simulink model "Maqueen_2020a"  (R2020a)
settings: Solver=VariableStepAuto  StartTime=0.0  StopTime=2  RelTol=1e-3
model workspace: external: MAT-File (data not in the file)
undefined symbols (not defined in the file or in its folder): deg, kg, m, mm, N, rad, s, smiData, X, Y, Z
libraries: sm_lib x459, fl_lib x12, nesl_utility x10
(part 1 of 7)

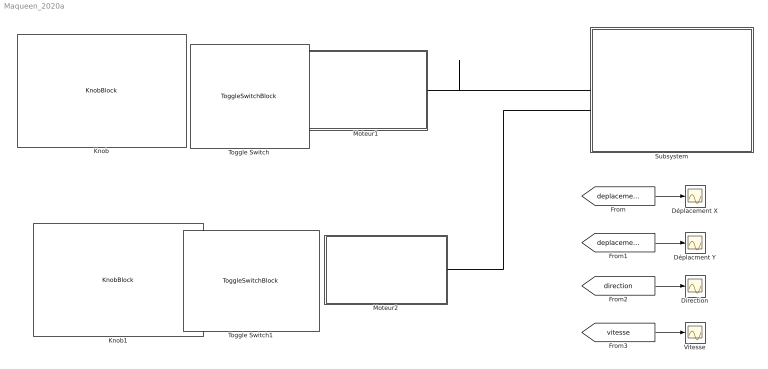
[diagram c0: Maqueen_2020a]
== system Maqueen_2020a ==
  Direction : Scope
  Déplacement X : Scope
  Déplacment Y : Scope
  Knob : KnobBlock  ScaleMax=255
  Knob1 : KnobBlock  ScaleMax=255
  Moteur1 : Subsystem
  Moteur2 : Subsystem
  Subsystem : Subsystem
  Toggle Switch : ToggleSwitchBlock
  Toggle Switch1 : ToggleSwitchBlock
  Vitesse : Scope
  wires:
  [deplacementX] -> Déplacement X/1
  [vitesse] -> Vitesse/1
  [direction] -> Direction/1
  [deplacementY] -> Déplacment Y/1
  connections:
  Moteur2/RConn1 -- Subsystem/LConn2
  Moteur1/RConn1 -- Subsystem/LConn1

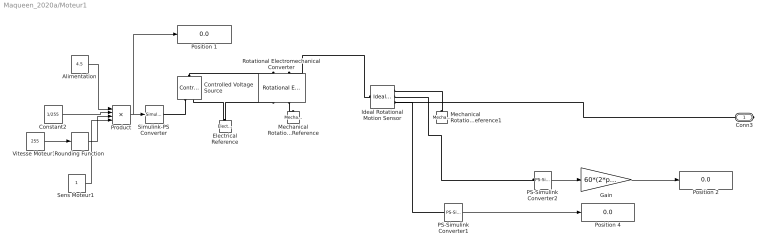
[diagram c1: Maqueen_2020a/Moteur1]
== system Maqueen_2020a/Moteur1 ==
  Alimentation : Constant  Value=4.5
  Constant2 : Constant  Value=1/255
  Controlled Voltage Source : fl_lib/Electrical/Electrical Sources/Controlled Voltage Source
  Electrical Reference : fl_lib/Electrical/Electrical Elements/Electrical Reference
  Gain : Gain  Gain=60*(2*pi)
  Ideal Rotational Motion Sensor : fl_lib/Mechanical/Mechanical Sensors/Ideal Rotational Motion Sensor  wrap_angle=simscape.enum.onoff.off  offset=0 rad
  Mechanical Rotational Reference : fl_lib/Mechanical/Rotational Elements/Mechanical Rotational Reference
  Mechanical Rotational Reference1 : fl_lib/Mechanical/Rotational Elements/Mechanical Rotational Reference
  PS-Simulink Converter1 : nesl_utility/PS-Simulink Converter  PhysicalDomain=network_engine_domain  SubClassName=ps_output  LeftPortType=input  RightPortType=output  PseudoPeriodic=off  Frequencies=[]  Unit=1  AffineConversion=off
  PS-Simulink Converter2 : nesl_utility/PS-Simulink Converter  PhysicalDomain=network_engine_domain  SubClassName=ps_output  LeftPortType=input  RightPortType=output  PseudoPeriodic=off  Frequencies=[]  Unit=1  AffineConversion=off
  Position 1 : Display
  Position 2 : Display
  Position 4 : Display
  Product : Product  Inputs=4
  Rotational Electromechanical Converter : fl_lib/Electrical/Electrical Elements/Rotational Electromechanical Converter  K=4.5/85.5 V/rpm  i_specify=off  i_priority=None  i=0 A  i_nominal_specify=off  i_nominal_unit=A  i_nominal_value=1  v_specify=off  v_priority=None  v=0 V  v_nominal_specify=off  v_nominal_unit=V  v_nominal_value=1  t_specify=off  t_priority=None  t=0 N*m  t_nominal_specify=off  t_nominal_unit=N*m  t_nominal_value=1  w_specify=off  w_priority=None  w=0 rad/s  w_nominal_specify=off  w_nominal_unit=rad/s  w_nominal_value=1
  Rounding Function : Rounding
  "Sens Moteur1 " : Constant
  Simulink-PS Converter : nesl_utility/Simulink-PS Converter  PhysicalDomain=network_engine_domain  SubClassName=ps_input  LeftPortType=input  RightPortType=output  PseudoPeriodic=off  Frequencies=[]  NoiseDistribution=none  NoiseParameters=[]  Unit=1  AffineConversion=off  FilteringAndDerivatives=provide  SimscapeFilterOrder=1  InputFilterTimeConstant=0.001  UdotUserProvided=0
  "Vitesse Moteur1 " : Constant  Value=255
  Conn3 : PMIOPort  Side=Right
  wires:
  "Sens Moteur1 "/1 -> Product/4
  Product/1 -> Position 1/1, Simulink-PS Converter/1
  "Vitesse Moteur1 "/1 -> Rounding Function/1
  Alimentation/1 -> Product/1
  Constant2/1 -> Product/2
  Rounding Function/1 -> Product/3
  PS-Simulink Converter2/1 -> Gain/1
  Gain/1 -> Position 2/1
  PS-Simulink Converter1/1 -> Position 4/1
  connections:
  Electrical Reference/LConn1 -- Rotational Electromechanical Converter/RConn1 -- Controlled Voltage Source/RConn2
  Rotational Electromechanical Converter/RConn2 -- Mechanical Rotational Reference/LConn1
  Ideal Rotational Motion Sensor/LConn1 -- Rotational Electromechanical Converter/LConn2
  Mechanical Rotational Reference1/LConn1 -- Ideal Rotational Motion Sensor/RConn1
  Controlled Voltage Source/RConn1 -- Simulink-PS Converter/RConn1
  Ideal Rotational Motion Sensor/RConn3 -- Conn3/RConn1 -- PS-Simulink Converter1/LConn1
  Controlled Voltage Source/LConn1 -- Rotational Electromechanical Converter/LConn1
  PS-Simulink Converter2/LConn1 -- Ideal Rotational Motion Sensor/RConn2

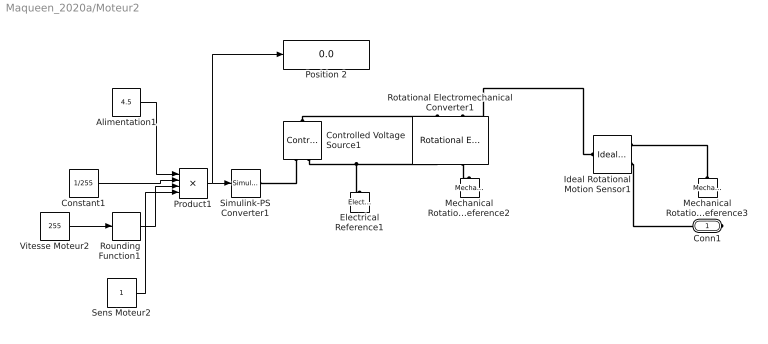
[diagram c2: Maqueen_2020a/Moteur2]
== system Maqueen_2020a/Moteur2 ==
  Alimentation1 : Constant  Value=4.5
  Constant1 : Constant  Value=1/255
  Controlled Voltage Source1 : fl_lib/Electrical/Electrical Sources/Controlled Voltage Source
  Electrical Reference1 : fl_lib/Electrical/Electrical Elements/Electrical Reference
  Ideal Rotational Motion Sensor1 : fl_lib/Mechanical/Mechanical Sensors/Ideal Rotational Motion Sensor  wrap_angle=simscape.enum.onoff.off  offset=0 rad
  Mechanical Rotational Reference2 : fl_lib/Mechanical/Rotational Elements/Mechanical Rotational Reference
  Mechanical Rotational Reference3 : fl_lib/Mechanical/Rotational Elements/Mechanical Rotational Reference
  Position 2 : Display
  Product1 : Product  Inputs=4
  Rotational Electromechanical Converter1 : fl_lib/Electrical/Electrical Elements/Rotational Electromechanical Converter  K=4.5/85.5 V/rpm  i_specify=off  i_priority=None  i=0 A  i_nominal_specify=off  i_nominal_unit=A  i_nominal_value=1  v_specify=off  v_priority=None  v=0 V  v_nominal_specify=off  v_nominal_unit=V  v_nominal_value=1  t_specify=off  t_priority=None  t=0 N*m  t_nominal_specify=off  t_nominal_unit=N*m  t_nominal_value=1  w_specify=off  w_priority=None  w=0 rad/s  w_nominal_specify=off  w_nominal_unit=rad/s  w_nominal_value=1
  Rounding Function1 : Rounding
  Sens Moteur2 : Constant
  Simulink-PS Converter1 : nesl_utility/Simulink-PS Converter  PhysicalDomain=network_engine_domain  SubClassName=ps_input  LeftPortType=input  RightPortType=output  PseudoPeriodic=off  Frequencies=[]  NoiseDistribution=none  NoiseParameters=[]  Unit=1  AffineConversion=off  FilteringAndDerivatives=provide  SimscapeFilterOrder=1  InputFilterTimeConstant=0.001  UdotUserProvided=0
  Vitesse Moteur2 : Constant  Value=255
  Conn1 : PMIOPort  Side=Right
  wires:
  Vitesse Moteur2/1 -> Rounding Function1/1
  Alimentation1/1 -> Product1/1
  Sens Moteur2/1 -> Product1/4
  Product1/1 -> Position 2/1, Simulink-PS Converter1/1
  Rounding Function1/1 -> Product1/3
  Constant1/1 -> Product1/2
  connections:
  Ideal Rotational Motion Sensor1/RConn3 -- Conn1/RConn1
  Controlled Voltage Source1/RConn1 -- Simulink-PS Converter1/RConn1
  Rotational Electromechanical Converter1/RConn2 -- Mechanical Rotational Reference2/LConn1
  Controlled Voltage Source1/RConn2 -- Rotational Electromechanical Converter1/RConn1 -- Electrical Reference1/LConn1
  Ideal Rotational Motion Sensor1/LConn1 -- Rotational Electromechanical Converter1/LConn2
  Mechanical Rotational Reference3/LConn1 -- Ideal Rotational Motion Sensor1/RConn1
  Controlled Voltage Source1/LConn1 -- Rotational Electromechanical Converter1/LConn1

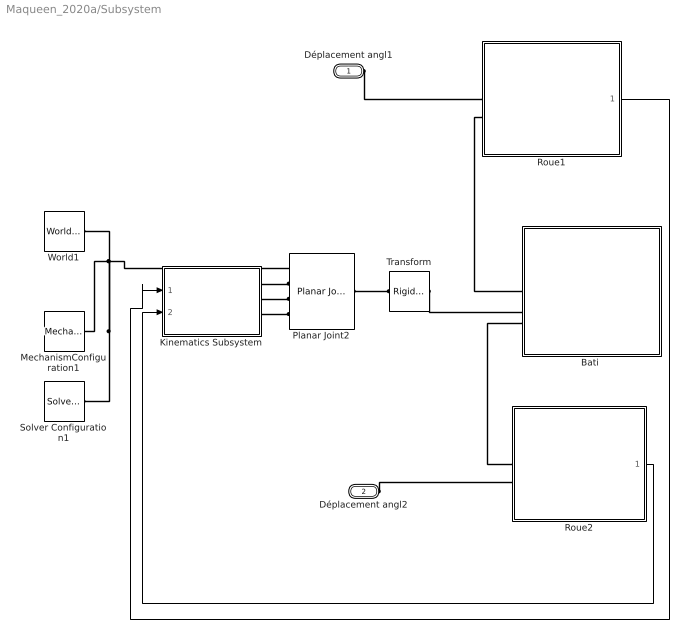
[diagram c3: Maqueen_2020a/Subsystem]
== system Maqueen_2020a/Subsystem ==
  "Bati " : Subsystem
  Kinematics Subsystem : Subsystem
  MechanismConfiguration1 : sm_lib/Utilities/Mechanism Configuration  UniformGravity=Constant  GravityVector=[0 0 -9.80665]  GravityUnits=m/s^2  LinearizationDelta=0.001
  Planar Joint2 : sm_lib/Joints/Planar Joint  JointMode=Normal  SenseConstraintForce=off  SenseConstraintForceX=off  SenseConstraintForceY=off  SenseConstraintForceZ=off  SenseConstraintTorque=off  SenseConstraintTorqueX=off  SenseConstraintTorqueY=off  SenseConstraintTorqueZ=off  SenseTotalForce=off  SenseTotalForceX=off  SenseTotalForceY=off  SenseTotalForceZ=off  SenseTotalTorque=off  SenseTotalTorqueX=off  SenseTotalTorqueY=off  SenseTotalTorqueZ=off  CompositeWrenchDir=FollowerOnBase  CompositeWrenchFrame=BaseFrame  PxEquilibriumPosition=0  PxEquilibriumPositionUnits=m  PxSpringStiffness=0  PxSpringStiffnessUnits=N/m  PxDampingCoefficient=0  PxDampingCoefficientUnits=N/(m/s)  PxTorqueActuationMode=ComputedTorque  PxMotionActuationMode=InputMotion  PxSensePosition=off  PxSenseVelocity=off  PxSenseAcceleration=off  PxSenseTorqueForce=off  PxSenseLowerLimitTorqueForce=off  PxSenseUpperLimitTorqueForce=off  PxLowerLimitSpecify=off  PxLowerLimitBound=-1  PxLowerLimitBoundUnits=m  PxLowerLimitStiffness=1e6  PxLowerLimitStiffnessUnits=N/m  PxLowerLimitDamping=1e3  PxLowerLimitDampingUnits=N/(m/s)  PxLowerLimitTransitionRegionWidth=1e-4  PxLowerLimitTransitionRegionWidthUnits=m  PxUpperLimitSpecify=off  PxUpperLimitBound=1  PxUpperLimitBoundUnits=m  PxUpperLimitStiffness=1e6  PxUpperLimitStiffnessUnits=N/m  PxUpperLimitDamping=1e3  PxUpperLimitDampingUnits=N/(m/s)  PxUpperLimitTransitionRegionWidth=1e-4  PxUpperLimitTransitionRegionWidthUnits=m  PxPositionTargetSpecify=off  PxPositionTargetPriority=High  PxPositionTargetValue=0  PxPositionTargetValueUnits=m  PxVelocityTargetSpecify=off  PxVelocityTargetPriority=High  PxVelocityTargetValue=0  PxVelocityTargetValueUnits=m/s  PyEquilibriumPosition=0  PyEquilibriumPositionUnits=m  PySpringStiffness=0  PySpringStiffnessUnits=N/m  PyDampingCoefficient=0  PyDampingCoefficientUnits=N/(m/s)  PyTorqueActuationMode=ComputedTorque  PyMotionActuationMode=InputMotion  PySensePosition=off  PySenseVelocity=off  PySenseAcceleration=off  PySenseTorqueForce=off  PySenseLowerLimitTorqueForce=off  PySenseUpperLimitTorqueForce=off  PyLowerLimitSpecify=off  PyLowerLimitBound=-1  PyLowerLimitBoundUnits=m  PyLowerLimitStiffness=1e6  PyLowerLimitStiffnessUnits=N/m  PyLowerLimitDamping=1e3  PyLowerLimitDampingUnits=N/(m/s)  PyLowerLimitTransitionRegionWidth=1e-4  PyLowerLimitTransitionRegionWidthUnits=m  PyUpperLimitSpecify=off  PyUpperLimitBound=1  PyUpperLimitBoundUnits=m  PyUpperLimitStiffness=1e6  PyUpperLimitStiffnessUnits=N/m  PyUpperLimitDamping=1e3  PyUpperLimitDampingUnits=N/(m/s)  PyUpperLimitTransitionRegionWidth=1e-4  PyUpperLimitTransitionRegionWidthUnits=m  PyPositionTargetSpecify=off  PyPositionTargetPriority=High  PyPositionTargetValue=0  PyPositionTargetValueUnits=m  PyVelocityTargetSpecify=off  PyVelocityTargetPriority=High  PyVelocityTargetValue=0  PyVelocityTargetValueUnits=m/s  RzEquilibriumPosition=0  RzEquilibriumPositionUnits=deg  RzSpringStiffness=0  RzSpringStiffnessUnits=N*m/deg  RzDampingCoefficient=0  RzDampingCoefficientUnits=N*m/(deg/s)  RzTorqueActuationMode=ComputedTorque  RzMotionActuationMode=InputMotion  RzSensePosition=off  RzSenseVelocity=off  RzSenseAcceleration=off  RzSenseTorqueForce=off  RzSenseLowerLimitTorqueForce=off  RzSenseUpperLimitTorqueForce=off  RzLowerLimitSpecify=off  RzLowerLimitBound=-90  RzLowerLimitBoundUnits=deg  RzLowerLimitStiffness=1e4  RzLowerLimitStiffnessUnits=N*m/deg  RzLowerLimitDamping=10  RzLowerLimitDampingUnits=N*m/(deg/s)  RzLowerLimitTransitionRegionWidth=0.1  RzLowerLimitTransitionRegionWidthUnits=deg  RzUpperLimitSpecify=off  RzUpperLimitBound=90  RzUpperLimitBoundUnits=deg  RzUpperLimitStiffness=1e4  RzUpperLimitStiffnessUnits=N*m/deg  RzUpperLimitDamping=10  RzUpperLimitDampingUnits=N*m/(deg/s)  RzUpperLimitTransitionRegionWidth=0.1  RzUpperLimitTransitionRegionWidthUnits=deg  RzPositionTargetSpecify=off  RzPositionTargetPriority=High  RzPositionTargetValue=0  RzPositionTargetValueUnits=deg  RzVelocityTargetSpecify=off  RzVelocityTargetPriority=High  RzVelocityTargetValue=0  RzVelocityTargetValueUnits=deg/s
  Roue1 : Subsystem
  Roue2 : Subsystem
  Solver Configuration1 : nesl_utility/Solver Configuration  PhysicalDomain=network_engine_domain  SubClassName=solver  LeftPortType=input  RightPortType=generic  Tones=[]  Harmonics=[]  SimulateNoise=off  Profile=off  UseLocalSampling=off  EnableSwitchedLinearOptims=on  FrequencyDomain=off  UseCCode=off  RelTol=0.001  AbsTol=1e-06  MinStep=1e-09  ToWorkspace=off  RevertToSquareIcSolve=off  NumHomotopyIterations=100  PhasorMode=off  PhasorModeNumHarmonics=1  DoDC=off  ResidualTolerance=1e-09  UseLocalSolver=off  LocalSolverChoice=NE_BACKWARD_EULER_ADVANCER  LocalSolverSampleTime=0.001  DoFixedCost=off  MaxNonlinIter=3  MaxModeIter=2  LinearAlgebra=Sparse  EquationFormulation=NE_TIME_EF  DelaysMemoryBudget=1024  AutomaticFiltering=on  FilteringTimeConstant=0.001  PartitionStorageMethod=AS_NEEDED  PartitionMemoryBudget=1024  PartitionMethod=FAST
  Transform : sm_lib/Frames and Transforms/Rigid Transform  TranslationMethod=Cartesian  TranslationStandardOffset=0  TranslationLengthUnit=mm  TranslationStandardAxis=+Z  TranslationCartesianOffset=smiData.RigidTransform(161).translation  TranslationROffset=0  TranslationROffsetUnits=m  TranslationZOffset=0  TranslationZOffsetUnits=m  TranslationThetaOffset=0  TranslationThetaOffsetUnits=deg  RotationMethod=ArbitraryAxis  RotationAngleUnits=rad  RotationStandardAxis=+Z  RotationAngle=smiData.RigidTransform(161).angle  RotationArbitraryAxis=smiData.RigidTransform(161).axis  FollAlignAxisA=+X  BaseAlignAxisA=+Y  FollAlignAxisB=+Y  BaseAlignAxisB=+Z  RotationSequenceAxes=FollowerAxes  RotationSequence=XYX  RotationSequenceAngles=[0 0 0]  RotationSequenceAnglesUnits=deg  RotationMatrix=[1 0 0; 0 1 0; 0 0 1]
  World1 : sm_lib/Frames and Transforms/World Frame
  Déplacement angl1 : PMIOPort  Side=Left
  Déplacement angl2 : PMIOPort  Port=2  Side=Left
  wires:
  Roue2/1(Out1) -> Kinematics Subsystem/2(w_r)
  Roue1/1(Out1) -> Kinematics Subsystem/1(w_l)
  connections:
  MechanismConfiguration1/RConn1 -- Solver Configuration1/RConn1 -- Planar Joint2/LConn1 -- World1/RConn1
  "Bati "/LConn1 -- Roue1/LConn2
  Transform/RConn1 -- "Bati "/LConn2
  "Bati "/LConn3 -- Roue2/LConn1
  Planar Joint2/RConn1 -- Transform/LConn1
  Kinematics Subsystem/RConn1 -- Planar Joint2/LConn2
  Kinematics Subsystem/RConn2 -- Planar Joint2/LConn3
  Kinematics Subsystem/RConn3 -- Planar Joint2/LConn4
  Déplacement angl2/RConn1 -- Roue2/LConn2
  Déplacement angl1/RConn1 -- Roue1/LConn1

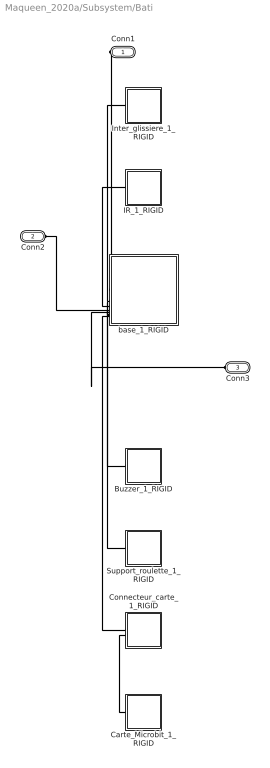
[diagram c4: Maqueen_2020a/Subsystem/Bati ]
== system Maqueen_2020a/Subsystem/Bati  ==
  Buzzer_1_RIGID : Subsystem
  Carte_Microbit_1_RIGID : Subsystem
  Connecteur_carte_1_RIGID : Subsystem
  IR_1_RIGID : Subsystem
  Inter_glissiere_1_RIGID : Subsystem
  Support_roulette_1_RIGID : Subsystem
  base_1_RIGID : Subsystem
  Conn1 : PMIOPort  Side=Left
  Conn2 : PMIOPort  Port=2  Side=Left
  Conn3 : PMIOPort  Port=3  Side=Left
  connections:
  base_1_RIGID/LConn1 -- Conn1/RConn1
  Support_roulette_1_RIGID/LConn1 -- base_1_RIGID/LConn7
  Connecteur_carte_1_RIGID/LConn1 -- base_1_RIGID/LConn8
  IR_1_RIGID/LConn1 -- base_1_RIGID/LConn3
  Carte_Microbit_1_RIGID/LConn1 -- Connecteur_carte_1_RIGID/LConn2
  Conn2/RConn1 -- base_1_RIGID/LConn4
  Inter_glissiere_1_RIGID/LConn1 -- base_1_RIGID/LConn2
  Buzzer_1_RIGID/LConn1 -- base_1_RIGID/LConn6
  base_1_RIGID/LConn5 -- Conn3/RConn1

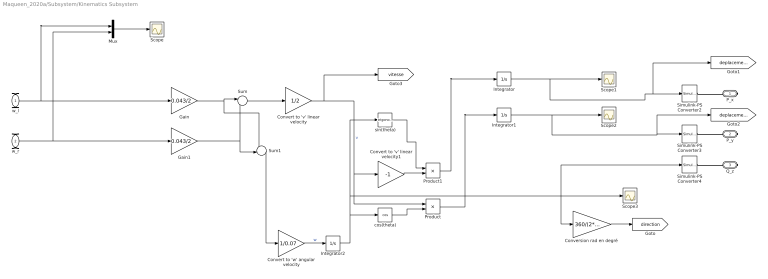
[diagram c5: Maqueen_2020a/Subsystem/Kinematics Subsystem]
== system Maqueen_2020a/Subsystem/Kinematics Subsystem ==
  w_l : Inport
  w_r : Inport  Port=2
  "Conversion rad en degré " : Gain  Gain=360/(2*pi)
  Convert to 'v' linear velocity : Gain  Gain=1/2
  Convert to 'v' linear velocity1 : Gain  Gain=-1
  Convert to 'w' angular velocity : Gain  Gain=1/0.07
  Gain : Gain  Gain=0.043/2
  Gain1 : Gain  Gain=0.043/2
  Integrator : Integrator
  Integrator1 : Integrator
  Integrator2 : Integrator
  Mux : Mux  Inputs=2
  Product : Product
  Product1 : Product
  Scope{,1..3} (4 alike) : Scope
  Simulink-PS Converter2 : nesl_utility/Simulink-PS Converter  PhysicalDomain=network_engine_domain  SubClassName=ps_input  LeftPortType=input  RightPortType=output  PseudoPeriodic=off  Frequencies=[]  NoiseDistribution=none  NoiseParameters=[]  Unit=1  AffineConversion=off  FilteringAndDerivatives=filter  SimscapeFilterOrder=2  InputFilterTimeConstant=0.01  UdotUserProvided=1
  Simulink-PS Converter3 : nesl_utility/Simulink-PS Converter  PhysicalDomain=network_engine_domain  SubClassName=ps_input  LeftPortType=input  RightPortType=output  PseudoPeriodic=off  Frequencies=[]  NoiseDistribution=none  NoiseParameters=[]  Unit=1  AffineConversion=off  FilteringAndDerivatives=filter  SimscapeFilterOrder=2  InputFilterTimeConstant=0.01  UdotUserProvided=1
  Simulink-PS Converter4 : nesl_utility/Simulink-PS Converter  PhysicalDomain=network_engine_domain  SubClassName=ps_input  LeftPortType=input  RightPortType=output  PseudoPeriodic=off  Frequencies=[]  NoiseDistribution=none  NoiseParameters=[]  Unit=1  AffineConversion=off  FilteringAndDerivatives=filter  SimscapeFilterOrder=2  InputFilterTimeConstant=0.01  UdotUserProvided=1
  Sum : Sum  Inputs=|++
  Sum1 : Sum  Inputs=-+|
  cos(theta) : Trigonometry  Operator=cos
  sin(theta) : Trigonometry
  P_x : PMIOPort  Side=Right
  P_y : PMIOPort  Port=2  Side=Right
  Q_z : PMIOPort  Port=3  Side=Right
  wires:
  Convert to 'v' linear velocity1/1 -> Product1/2
  Mux/1 -> Scope/1
  Product/1 -> Integrator1/1
  Product1/1 -> Integrator/1
  w_r/1 -> Gain1/1, Mux/2
  w_l/1 -> Gain/1, Mux/1
  Convert to 'v' linear velocity/1 -> [vitesse], Product/1, Convert to 'v' linear velocity1/1  "v"
  Sum1/1 -> Convert to 'w' angular velocity/1
  cos(theta)/1 -> Product/2
  sin(theta)/1 -> Product1/1
  Integrator2/1 -> cos(theta)/1, sin(theta)/1, Scope3/1, "Conversion rad en degré "/1, Simulink-PS Converter4/1
  Convert to 'w' angular velocity/1 -> Integrator2/1  "w"
  Integrator1/1 -> Scope2/1, [deplacementY], Simulink-PS Converter3/1
  Sum/1 -> Convert to 'v' linear velocity/1
  Gain/1 -> Sum/1, Sum1/1
  Gain1/1 -> Sum1/2, Sum/2
  "Conversion rad en degré "/1 -> [direction]
  Integrator/1 -> Scope1/1, [deplacementX], Simulink-PS Converter2/1
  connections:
  Simulink-PS Converter3/RConn1 -- P_y/RConn1
  Simulink-PS Converter2/RConn1 -- P_x/RConn1
  Simulink-PS Converter4/RConn1 -- Q_z/RConn1

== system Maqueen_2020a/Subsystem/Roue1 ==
  PS-Simulink Converter3 : nesl_utility/PS-Simulink Converter  PhysicalDomain=network_engine_domain  SubClassName=ps_output  LeftPortType=input  RightPortType=output  PseudoPeriodic=off  Frequencies=[]  Unit=1  AffineConversion=off
  Revolute : sm_lib/Joints/Revolute Joint  JointMode=Normal  SenseConstraintForce=off  SenseConstraintForceX=off  SenseConstraintForceY=off  SenseConstraintForceZ=off  SenseConstraintTorque=off  SenseConstraintTorqueX=off  SenseConstraintTorqueY=off  SenseConstraintTorqueZ=off  SenseTotalForce=off  SenseTotalForceX=off  SenseTotalForceY=off  SenseTotalForceZ=off  SenseTotalTorque=off  SenseTotalTorqueX=off  SenseTotalTorqueY=off  SenseTotalTorqueZ=off  CompositeWrenchDir=FollowerOnBase  CompositeWrenchFrame=BaseFrame  EquilibriumPosition=0  EquilibriumPositionUnits=rad  SpringStiffness=0  SpringStiffnessUnits=N*m/rad  DampingCoefficient=0  DampingCoefficientUnits=N*m/(rad/s)  TorqueActuationMode=ComputedTorque  MotionActuationMode=InputMotion  SensePosition=off  SenseVelocity=on  SenseAcceleration=off  SenseTorqueForce=off  SenseLowerLimitTorqueForce=off  SenseUpperLimitTorqueForce=off  LowerLimitSpecify=off  LowerLimitBound=-90  LowerLimitBoundUnits=deg  LowerLimitStiffness=1e4  LowerLimitStiffnessUnits=N*m/deg  LowerLimitDamping=10  LowerLimitDampingUnits=N*m/(deg/s)  LowerLimitTransitionRegionWidth=0.1  LowerLimitTransitionRegionWidthUnits=deg  UpperLimitSpecify=off  UpperLimitBound=90  UpperLimitBoundUnits=deg  UpperLimitStiffness=1e4  UpperLimitStiffnessUnits=N*m/deg  UpperLimitDamping=10  UpperLimitDampingUnits=N*m/(deg/s)  UpperLimitTransitionRegionWidth=0.1  UpperLimitTransitionRegionWidthUnits=deg  PositionTargetSpecify=on  PositionTargetPriority=Low  PositionTargetValue=smiData.RevoluteJoint(1).Rz.Pos  PositionTargetValueUnits=deg  VelocityTargetSpecify=off  VelocityTargetPriority=High  VelocityTargetValue=0  VelocityTargetValueUnits=deg/s
  Roue_2_RIGID : Subsystem
  bloc_moteur_1_RIGID : Subsystem
  Conn1 : PMIOPort  Side=Left
  Conn2 : PMIOPort  Port=2  Side=Left
  Out1 : Outport  VectorParamsAs1DForOutWhenUnconnected=off
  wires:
  PS-Simulink Converter3/1 -> Out1/1
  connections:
  Revolute/LConn2 -- Conn1/RConn1
  Revolute/LConn1 -- Roue_2_RIGID/RConn1
  Revolute/RConn1 -- bloc_moteur_1_RIGID/LConn1
  Conn2/RConn1 -- bloc_moteur_1_RIGID/LConn2
  Revolute/RConn2 -- PS-Simulink Converter3/LConn1

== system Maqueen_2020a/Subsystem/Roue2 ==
  PS-Simulink Converter1 : nesl_utility/PS-Simulink Converter  PhysicalDomain=network_engine_domain  SubClassName=ps_output  LeftPortType=input  RightPortType=output  PseudoPeriodic=off  Frequencies=[]  Unit=1  AffineConversion=off
  Revolute1 : sm_lib/Joints/Revolute Joint  JointMode=Normal  SenseConstraintForce=off  SenseConstraintForceX=off  SenseConstraintForceY=off  SenseConstraintForceZ=off  SenseConstraintTorque=off  SenseConstraintTorqueX=off  SenseConstraintTorqueY=off  SenseConstraintTorqueZ=off  SenseTotalForce=off  SenseTotalForceX=off  SenseTotalForceY=off  SenseTotalForceZ=off  SenseTotalTorque=off  SenseTotalTorqueX=off  SenseTotalTorqueY=off  SenseTotalTorqueZ=off  CompositeWrenchDir=FollowerOnBase  CompositeWrenchFrame=BaseFrame  EquilibriumPosition=0  EquilibriumPositionUnits=rad  SpringStiffness=0  SpringStiffnessUnits=N*m/rad  DampingCoefficient=0  DampingCoefficientUnits=N*m/(rad/s)  TorqueActuationMode=ComputedTorque  MotionActuationMode=InputMotion  SensePosition=off  SenseVelocity=on  SenseAcceleration=off  SenseTorqueForce=off  SenseLowerLimitTorqueForce=off  SenseUpperLimitTorqueForce=off  LowerLimitSpecify=off  LowerLimitBound=-90  LowerLimitBoundUnits=deg  LowerLimitStiffness=1e4  LowerLimitStiffnessUnits=N*m/deg  LowerLimitDamping=10  LowerLimitDampingUnits=N*m/(deg/s)  LowerLimitTransitionRegionWidth=0.1  LowerLimitTransitionRegionWidthUnits=deg  UpperLimitSpecify=off  UpperLimitBound=90  UpperLimitBoundUnits=deg  UpperLimitStiffness=1e4  UpperLimitStiffnessUnits=N*m/deg  UpperLimitDamping=10  UpperLimitDampingUnits=N*m/(deg/s)  UpperLimitTransitionRegionWidth=0.1  UpperLimitTransitionRegionWidthUnits=deg  PositionTargetSpecify=on  PositionTargetPriority=Low  PositionTargetValue=smiData.RevoluteJoint(2).Rz.Pos  PositionTargetValueUnits=deg  VelocityTargetSpecify=off  VelocityTargetPriority=High  VelocityTargetValue=0  VelocityTargetValueUnits=deg/s
  Roue_1 : Subsystem
  bloc_moteur_2_RIGID : Subsystem
  Conn1 : PMIOPort  Side=Left
  Conn2 : PMIOPort  Port=2  Side=Left
  Out1 : Outport  VectorParamsAs1DForOutWhenUnconnected=off
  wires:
  PS-Simulink Converter1/1 -> Out1/1
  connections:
  Conn1/RConn1 -- bloc_moteur_2_RIGID/LConn1
  Revolute1/LConn1 -- Roue_1/RConn1
  Revolute1/RConn1 -- bloc_moteur_2_RIGID/LConn2
  Revolute1/LConn2 -- Conn2/RConn1
  PS-Simulink Converter1/LConn1 -- Revolute1/RConn2

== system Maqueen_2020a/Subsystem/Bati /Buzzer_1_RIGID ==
  ReferenceFrame : sm_lib/Frames and Transforms/Reference Frame
  Solid : sm_lib/Body Elements/File Solid  ExtGeomFileName=Buzzer_Defaut_sldprt.STL  UnitType=Custom  ExtGeomFileUnits=mm  StepReaderType=HEX  ExportConvexHullGeometry=off  InertiaType=Custom  Mass=smiData.Solid(4).mass  MassUnits=kg  CenterOfMass=smiData.Solid(4).CoM  CenterOfMassUnits=mm  MomentsOfInertia=smiData.Solid(4).MoI  MomentsOfInertiaUnits=kg*mm^2  ProductsOfInertia=smiData.Solid(4).PoI  ProductsOfInertiaUnits=kg*mm^2  BasedOnType=Density  Density=1000  DensityUnits=kg/m^3  DoExposeReferenceFrame=on  SerializedFrames=<Frames/>  GraphicType=FromGeometry  MarkerShape=Sphere  MarkerSize=10  GraphicVisPropType=SimpleVisualProperties  GraphicDiffuseColor=smiData.Solid(4).color  GraphicSpecularColor=[0.5 0.5 0.5 1.0]  GraphicAmbientColor=[0.15 0.15 0.15 1.0]  GraphicEmissiveColor=[0.0 0.0 0.0 1.0]  GraphicShininess=75  GraphicOpacity=smiData.Solid(4).opacity
  Transform : sm_lib/Frames and Transforms/Rigid Transform  TranslationMethod=Cartesian  TranslationStandardOffset=0  TranslationLengthUnit=mm  TranslationStandardAxis=+Z  TranslationCartesianOffset=smiData.RigidTransform(14).translation  TranslationROffset=0  TranslationROffsetUnits=m  TranslationZOffset=0  TranslationZOffsetUnits=m  TranslationThetaOffset=0  TranslationThetaOffsetUnits=deg  RotationMethod=ArbitraryAxis  RotationAngleUnits=rad  RotationStandardAxis=+Z  RotationAngle=smiData.RigidTransform(14).angle  RotationArbitraryAxis=smiData.RigidTransform(14).axis  FollAlignAxisA=+X  BaseAlignAxisA=+Y  FollAlignAxisB=+Y  BaseAlignAxisB=+Z  RotationSequenceAxes=FollowerAxes  RotationSequence=XYX  RotationSequenceAngles=[0 0 0]  RotationSequenceAnglesUnits=deg  RotationMatrix=[1 0 0; 0 1 0; 0 0 1]
  F : PMIOPort  Side=Left
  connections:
  ReferenceFrame/RConn1 -- Solid/RConn1 -- Transform/LConn1
  Transform/RConn1 -- F/RConn1
